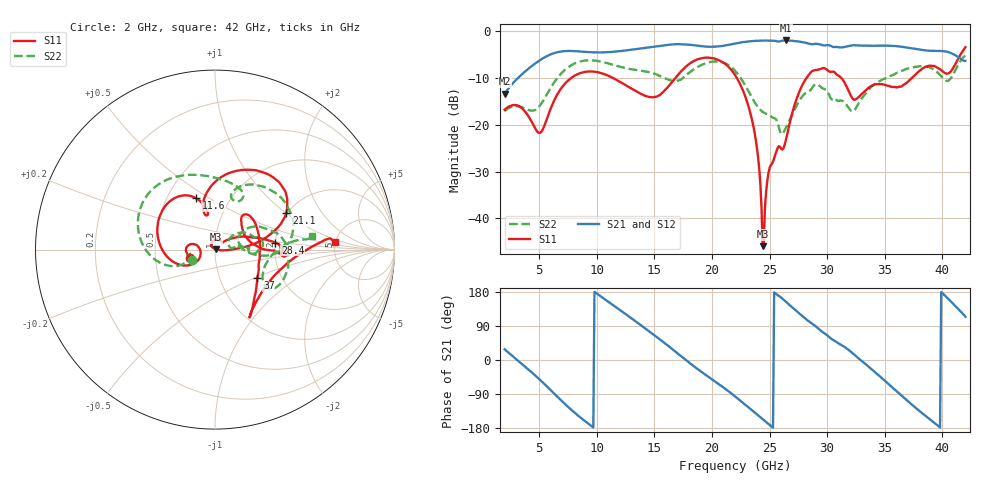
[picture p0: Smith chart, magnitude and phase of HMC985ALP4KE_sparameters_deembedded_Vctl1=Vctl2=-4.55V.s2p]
!s2p File: Measurements: S11, S21, S12, S22
# GHz S dB R 50.0
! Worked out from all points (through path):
!   401 points, 2 GHz to 42 GHz, reference 50 ohm
!   highest |S21| = -2.06 dB at 26.4 GHz (marker M1); lowest = -13.4 dB at 2 GHz (marker M2)
!   lowest |S11| = -45.9 dB at 24.4 GHz (marker M3), VSWR 1.01, Z = 50.5 + j0.168 ohm
!   |S11| at or under -10 dB: start of sweep to 7.818 GHz; 22.14 GHz to 28.23 GHz (6.083 GHz wide, 24.2 % of centre); 31.2 GHz to 37.38 GHz (6.179 GHz wide, 18 % of centre)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
!   |S22| runs from -22.0 to -5.3 dB; largest |S21 - S12| = 0.00066
!   S11 on the Smith chart (normalised r, x): 2 GHz: 0.76, -0.07; 11.6 GHz: 0.70, +0.44; 21.1 GHz: 1.97, +1.01; 28.4 GHz: 2.00, +0.18; 37 GHz: 1.51, -0.53; 42 GHz: 4.91, +0.74
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2  -16.84 -161.8  -13.44 28.2  -13.44 28.2  -17.14 -155.6
5  -21.78 -173.1  -6.38 -50.2  -6.38 -50.2  -16.14 -160.1
6.3  -14.87 -150.6  -4.76 -88.4  -4.76 -88.4  -11.01 -161.8
8.7  -8.93 150.2  -4.44 -154.7  -4.44 -154.7  -6.46 151.1
11.6  -10.32 110.2  -4.45 140.8  -4.45 140.8  -7.38 103.3
13.6  -13.15 101.3  -3.85 97.0  -3.85 97.0  -8.42 75.5
15.4  -13.79 106.2  -3.25 56.2  -3.25 56.2  -9.54 62.0
17.9  -7.30 80.0  -2.94 -3.9  -2.95 -3.9  -9.17 72.0
21.1  -6.99 27.4  -3.15 -74.8  -3.15 -74.7  -6.88 15.7
22  -9.40 16.8  -2.71 -96.0  -2.71 -95.9  -8.50 0.3
23.6  -20.41 0.4  -2.18 -135.7  -2.18 -135.7  -14.80 -4.2
24  -26.96 -5.4  -2.11 -145.7  -2.11 -145.7  -16.32 1.4
24.4  -45.92 19.2  -2.09 -155.8  -2.08 -155.8  -17.29 7.4
25.1  -28.69 124.8  -2.12 -173.6  -2.12 -173.6  -18.17 10.9
26.4  -23.48 41.6  -2.06 154.2  -2.06 154.2  -20.81 33.2
28.4  -9.40 6.6  -2.72 102.1  -2.73 102.1  -12.87 18.0
28.7  -8.58 1.6  -2.86 95.9  -2.87 95.9  -12.18 16.1
32.5  -14.57 32.7  -3.10 10.1  -3.10 10.2  -16.47 28.1
35.4  -11.79 18.7  -3.18 -65.3  -3.18 -65.3  -9.77 19.2
37  -10.88 -34.1  -3.60 -108.5  -3.60 -108.4  -8.06 4.6
39.8  -8.21 -57.1  -4.30 -178.2  -4.29 -178.2  -9.39 -35.5
42  -3.50 3.6  -6.41 114.1  -6.42 114.1  -5.25 8.1
